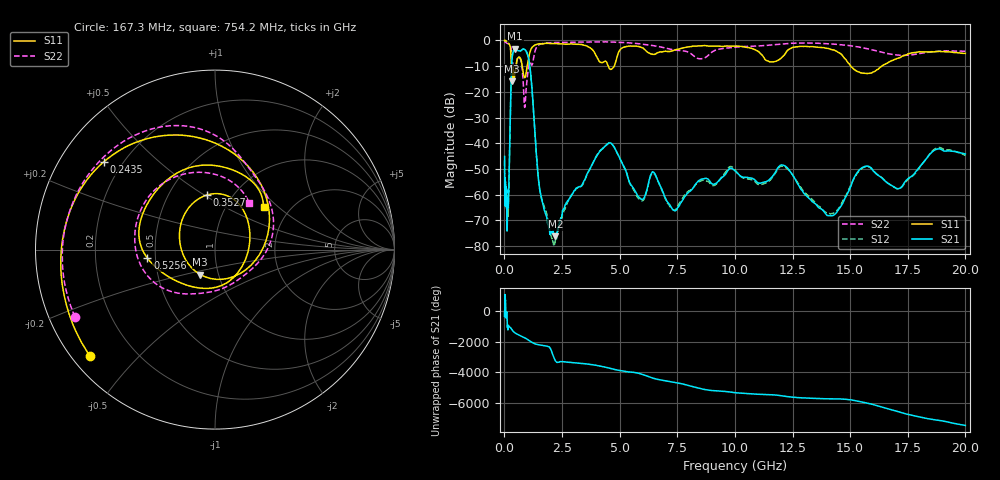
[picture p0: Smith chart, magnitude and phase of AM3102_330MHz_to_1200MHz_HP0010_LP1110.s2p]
! Date/Time: Tue, Sep 11, 2018 5:11 PM
! Network Analyzer: Agilent Technologies E8362B Rev: A.07.50.63
! Sweep from 0.010 to 20.000 GHz, 1601 Points, Sweep Type: LOG
! Power Supply: 4.949 V, 0.001 A
# Hz S DB R 50
!freq MagS11 AngS11 MagS21 AngS21 MagS12 AngS12 MagS22 AngS22
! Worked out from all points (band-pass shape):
!   1601 points, 10 MHz to 20 GHz, reference 50 ohm
!   highest |S21| = -3.16 dB at 473.4 MHz (marker M1); lowest = -76.3 dB at 2.217 GHz (marker M2)
!   |S21| within 3 dB of the highest: 342.6 MHz to 1.027 GHz (684.6 MHz wide, 100 % of centre)
!   lowest |S11| = -15.8 dB at 319.2 MHz (marker M3), VSWR 1.38, Z = 40.9 - j11.7 ohm
!   |S11| at or under -10 dB: 772.1 MHz to 988 MHz (215.9 MHz wide, 24.5 % of centre); 4.508 GHz to 4.765 GHz (256.5 MHz wide, 5.53 % of centre); 15.03 GHz to 16.38 GHz (1.348 GHz wide, 8.59 % of centre)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
!   |S22| runs from -26.1 to -0.3 dB; largest |S21 - S12| = 0.012
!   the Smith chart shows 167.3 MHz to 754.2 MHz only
!   S11 on the Smith chart (normalised r, x): 167.3 MHz: 0.05, -0.37; 243.5 MHz: 0.13, +0.34; 352.7 MHz: 0.76, +0.51; 525.6 MHz: 0.45, -0.05; 754.2 MHz: 1.48, +0.81
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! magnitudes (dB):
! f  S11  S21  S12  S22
! 10 MHz  0.0  -45.2  -46.8  -0.3
! 35.55 MHz  0.0  -62.1  -60.6  -0.6
! 91.5 MHz  -0.2  -58.5  -65.6  -1.0
! 126.4 MHz  -0.4  -71.9  -62.4  -1.1
! 167.3 MHz  -0.8  -65.0  -67.4  -1.3
! 243.5 MHz  -2.1  -36.1  -36.1  -1.8
! 319.2 MHz  -15.8  -8.5  -8.5  -5.5
! 352.7 MHz  -10.2  -5.6  -5.7  -7.8
! 447.2 MHz  -13.9  -3.2  -3.3  -13.1
! 473.4 MHz  -12.6  -3.2  -3.2  -12.0
! 525.6 MHz  -8.4  -3.5  -3.6  -8.6
! 754.2 MHz  -8.9  -3.7  -3.7  -9.8
! 882.2 MHz  -14.5  -3.5  -3.6  -26.1
! 1.103 GHz  -4.8  -10.0  -9.9  -8.5
! 1.59 GHz  -1.3  -60.4  -60.9  -1.3
! 2.217 GHz  -1.2  -76.3  -77.6  -0.8
! 4.457 GHz  -8.9  -40.5  -40.4  -0.5
! 5.652 GHz  -2.2  -58.3  -58.9  -1.1
! 7.41 GHz  -3.6  -66.3  -66.1  -3.7
! 12.09 GHz  -6.1  -48.6  -49.0  -1.3
! 14.14 GHz  -3.4  -68.2  -67.5  -1.3
! 20 GHz  -5.0  -44.2  -44.8  -4.2
